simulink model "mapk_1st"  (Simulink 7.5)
settings: Solver=ode45  StartTime=0.0  StopTime=1000  FixedStep=0.001  RelTol=1e-3
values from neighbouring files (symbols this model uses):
  k = load('parameter.txt', '-ascii')    [mapk_steering.m]
  x = xis+deltax    [mapk_steering.m]

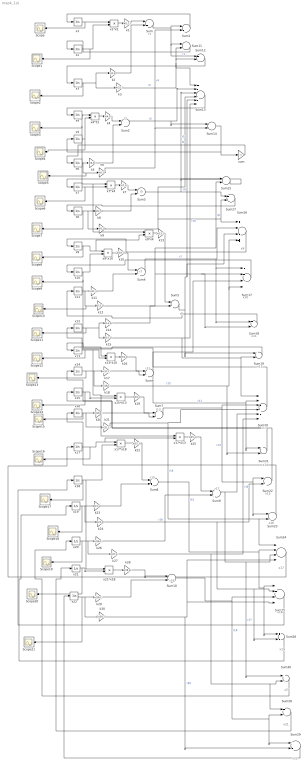
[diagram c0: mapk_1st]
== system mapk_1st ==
  note: r3
  note: r5
  note: r7
  note: r9
  note: r11
  note: r13
  note: r15
  note: r17
  note: r19
  note: x9
  note: x10
  note: x11
  note: x12
  note: x13
  note: x14
  note: x15
  note: x16
  note: x17
  note: x18
  note: x19
  note: x20
  note: x21
  note: x22
  note: r1
  Scope{,1..21} (22 alike) : Scope
  Sum{,2..10} (10 alike) : Sum  Inputs=|+-  OutDataType=fixdt(1, 16)  OutScaling=2^0
  Sum{1,11,14..15} (4 alike) : Sum  Inputs=|-+  OutDataType=fixdt(1, 16)  OutScaling=2^0
  Sum{12,18..19,21,23,26..30} (10 alike) : Sum  Inputs=+-  OutDataType=fixdt(1, 16)  OutScaling=2^0
  Sum13 : Sum  Inputs=+--+-+  OutDataType=fixdt(1, 16)  OutScaling=2^0
  Sum16 : Sum  Inputs=+--+  OutDataType=fixdt(1, 16)  OutScaling=2^0
  Sum17 : Sum  Inputs=-+-+  OutDataType=fixdt(1, 16)  OutScaling=2^0
  Sum20 : Sum  Inputs=+--+-+  OutDataType=fixdt(1, 16)  OutScaling=2^0
  Sum22 : Sum  Inputs=-+  OutDataType=fixdt(1, 16)  OutScaling=2^0
  Sum24 : Sum  Inputs=+--+  OutDataType=fixdt(1, 16)  OutScaling=2^0
  Sum25 : Sum  Inputs=-+-+  OutDataType=fixdt(1, 16)  OutScaling=2^0
  k1 : Gain  Gain=k(1,1)  ParameterDataType=fixdt(1, 16)  ParameterScaling=2^0  OutDataType=fixdt(1, 16)  OutScaling=2^0
  k10 : Gain  Gain=k(10,1)  ParameterDataType=fixdt(1, 16)  ParameterScaling=2^0  OutDataType=fixdt(1, 16)  OutScaling=2^0
  k11 : Gain  Gain=k(11,1)  ParameterDataType=fixdt(1, 16)  ParameterScaling=2^0  OutDataType=fixdt(1, 16)  OutScaling=2^0
  k12 : Gain  Gain=k(12,1)  ParameterDataType=fixdt(1, 16)  ParameterScaling=2^0  OutDataType=fixdt(1, 16)  OutScaling=2^0
  k13 : Gain  Gain=k(13,1)  ParameterDataType=fixdt(1, 16)  ParameterScaling=2^0  OutDataType=fixdt(1, 16)  OutScaling=2^0
  k14 : Gain  Gain=k(14,1)  ParameterDataType=fixdt(1, 16)  ParameterScaling=2^0  OutDataType=fixdt(1, 16)  OutScaling=2^0
  k15 : Gain  Gain=k(15,1)  ParameterDataType=fixdt(1, 16)  ParameterScaling=2^0  OutDataType=fixdt(1, 16)  OutScaling=2^0
  k16 : Gain  Gain=k(16,1)  ParameterDataType=fixdt(1, 16)  ParameterScaling=2^0  OutDataType=fixdt(1, 16)  OutScaling=2^0
  k17 : Gain  Gain=k(17,1)  ParameterDataType=fixdt(1, 16)  ParameterScaling=2^0  OutDataType=fixdt(1, 16)  OutScaling=2^0
  k18 : Gain  Gain=k(18,1)  ParameterDataType=fixdt(1, 16)  ParameterScaling=2^0  OutDataType=fixdt(1, 16)  OutScaling=2^0
  k19 : Gain  Gain=k(19,1)  ParameterDataType=fixdt(1, 16)  ParameterScaling=2^0  OutDataType=fixdt(1, 16)  OutScaling=2^0
  k2 : Gain  Gain=k(2,1)  ParameterDataType=fixdt(1, 16)  ParameterScaling=2^0  OutDataType=fixdt(1, 16)  OutScaling=2^0
  k20 : Gain  Gain=k(20,1)  ParameterDataType=fixdt(1, 16)  ParameterScaling=2^0  OutDataType=fixdt(1, 16)  OutScaling=2^0
  k21 : Gain  Gain=k(21,1)  ParameterDataType=fixdt(1, 16)  ParameterScaling=2^0  OutDataType=fixdt(1, 16)  OutScaling=2^0
  k22 : Gain  Gain=k(22,1)  ParameterDataType=fixdt(1, 16)  ParameterScaling=2^0  OutDataType=fixdt(1, 16)  OutScaling=2^0
  k23 : Gain  Gain=k(23,1)  ParameterDataType=fixdt(1, 16)  ParameterScaling=2^0  OutDataType=fixdt(1, 16)  OutScaling=2^0
  k24 : Gain  Gain=k(24,1)  ParameterDataType=fixdt(1, 16)  ParameterScaling=2^0  OutDataType=fixdt(1, 16)  OutScaling=2^0
  k25 : Gain  Gain=k(25,1)  ParameterDataType=fixdt(1, 16)  ParameterScaling=2^0  OutDataType=fixdt(1, 16)  OutScaling=2^0
  k26 : Gain  Gain=k(26,1)  ParameterDataType=fixdt(1, 16)  ParameterScaling=2^0  OutDataType=fixdt(1, 16)  OutScaling=2^0
  k27 : Gain  Gain=k(27,1)  ParameterDataType=fixdt(1, 16)  ParameterScaling=2^0  OutDataType=fixdt(1, 16)  OutScaling=2^0
  k28 : Gain  Gain=k(28,1)  ParameterDataType=fixdt(1, 16)  ParameterScaling=2^0  OutDataType=fixdt(1, 16)  OutScaling=2^0
  k29 : Gain  Gain=k(29,1)  ParameterDataType=fixdt(1, 16)  ParameterScaling=2^0  OutDataType=fixdt(1, 16)  OutScaling=2^0
  k3 : Gain  Gain=k(3,1)  ParameterDataType=fixdt(1, 16)  ParameterScaling=2^0  OutDataType=fixdt(1, 16)  OutScaling=2^0
  k30 : Gain  Gain=k(30,1)  ParameterDataType=fixdt(1, 16)  ParameterScaling=2^0  OutDataType=fixdt(1, 16)  OutScaling=2^0
  k4 : Gain  Gain=k(4,1)  ParameterDataType=fixdt(1, 16)  ParameterScaling=2^0  OutDataType=fixdt(1, 16)  OutScaling=2^0
  k5 : Gain  Gain=k(5,1)  ParameterDataType=fixdt(1, 16)  ParameterScaling=2^0  OutDataType=fixdt(1, 16)  OutScaling=2^0
  k6 : Gain  Gain=k(6,1)  ParameterDataType=fixdt(1, 16)  ParameterScaling=2^0  OutDataType=fixdt(1, 16)  OutScaling=2^0
  k7 : Gain  Gain=k(7,1)  ParameterDataType=fixdt(1, 16)  ParameterScaling=2^0  OutDataType=fixdt(1, 16)  OutScaling=2^0
  k8 : Gain  Gain=k(8,1)  ParameterDataType=fixdt(1, 16)  ParameterScaling=2^0  OutDataType=fixdt(1, 16)  OutScaling=2^0
  k9 : Gain  Gain=k(9,1)  ParameterDataType=fixdt(1, 16)  ParameterScaling=2^0  OutDataType=fixdt(1, 16)  OutScaling=2^0
  sum : Gain  Gain=-1  ParameterDataType=fixdt(1, 16)  ParameterScaling=2^0  OutDataType=fixdt(1, 16)  OutScaling=2^0
  x1 : Integrator  InitialCondition=x(1,1)  LimitOutput=on  LowerSaturationLimit=0
  x1*x2 : Product  OutDataType=fixdt(1, 16)  OutScaling=2^0
  x10 : Integrator  InitialCondition=x(10,1)  LimitOutput=on  LowerSaturationLimit=0
  x11 : Integrator  InitialCondition=x(11,1)  LimitOutput=on  LowerSaturationLimit=0
  x12 : Integrator  InitialCondition=x(12,1)  LimitOutput=on  LowerSaturationLimit=0
  x13 : Integrator  InitialCondition=x(13,1)  LimitOutput=on  LowerSaturationLimit=0
  x13*x10 : Product  OutDataType=fixdt(1, 16)  OutScaling=2^0
  x14 : Integrator  InitialCondition=x(14,1)  LimitOutput=on  LowerSaturationLimit=0
  x15 : Integrator  InitialCondition=x(15,1)  LimitOutput=on  LowerSaturationLimit=0
  x15*x13 : Product  OutDataType=fixdt(1, 16)  OutScaling=2^0
  x16 : Integrator  InitialCondition=x(16,1)  LimitOutput=on  LowerSaturationLimit=0
  x17 : Integrator  InitialCondition=x(17,1)  LimitOutput=on  LowerSaturationLimit=0
  x17*x13 : Product  OutDataType=fixdt(1, 16)  OutScaling=2^0
  x17*x18 : Product  OutDataType=fixdt(1, 16)  OutScaling=2^0
  x18 : Integrator  InitialCondition=x(18,1)  LimitOutput=on  LowerSaturationLimit=0
  x19 : Integrator  InitialCondition=x(19,1)  LimitOutput=on  LowerSaturationLimit=0
  x2 : Integrator  InitialCondition=x(2,1)  LimitOutput=on  LowerSaturationLimit=0
  x20 : Integrator  InitialCondition=x(20,1)  LimitOutput=on  LowerSaturationLimit=0
  x21 : Integrator  InitialCondition=x(21,1)  LimitOutput=on  LowerSaturationLimit=0
  x21*x18 : Product  OutDataType=fixdt(1, 16)  OutScaling=2^0
  x22 : Integrator  InitialCondition=x(22,1)  LimitOutput=on  LowerSaturationLimit=0  ZeroCross=off
  x3 : Integrator  InitialCondition=x(3,1)  LimitOutput=on  LowerSaturationLimit=0
  x4 : Integrator  InitialCondition=x(4,1)  LimitOutput=on  LowerSaturationLimit=0
  x4*51 : Product  OutDataType=fixdt(1, 16)  OutScaling=2^0
  x5 : Integrator  InitialCondition=x(5,1)  LimitOutput=on  LowerSaturationLimit=0
  x6 : Integrator  InitialCondition=x(6,1)  LimitOutput=on  LowerSaturationLimit=0
  x7 : Integrator  InitialCondition=x(7,1)  LimitOutput=on  LowerSaturationLimit=0
  x7*x4 : Product  OutDataType=fixdt(1, 16)  OutScaling=2^0
  x8 : Integrator  InitialCondition=x(8,1)  LimitOutput=on  LowerSaturationLimit=0
  x9 : Integrator  InitialCondition=x(9,1)  LimitOutput=on  LowerSaturationLimit=0
  x9*x10 : Product  OutDataType=fixdt(1, 16)  OutScaling=2^0
  x9*x4 : Product  OutDataType=fixdt(1, 16)  OutScaling=2^0
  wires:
  x2/1 -> Scope1/1, x1*x2/2
  x3/1 -> k2/1, k3/1, Scope2/1
  k2/1 -> Sum/2
  x4/1 -> x4*51/1, x7*x4/1, x9*x4/1, Scope3/1
  x5/1 -> x4*51/2, Scope4/1
  x4*51/1 -> k4/1
  x6/1 -> k6/1, Scope5/1, k5/1
  k4/1 -> Sum2/1
  k5/1 -> Sum2/2
  x7/1 -> x7*x4/2, Scope6/1
  x7*x4/1 -> k7/1
  x8/1 -> k8/1, k9/1, Scope7/1
  k7/1 -> Sum3/1
  k8/1 -> Sum3/2
  x9/1 -> x9*x10/1, x9*x4/2, Scope8/1
  x10/1 -> x9*x10/2, x13*x10/1, Scope9/1
  x9*x10/1 -> k10/1
  x11/1 -> k11/1, k12/1, Scope10/1
  k10/1 -> Sum4/1
  k11/1 -> Sum4/2
  x9*x4/1 -> k13/1
  k13/1 -> Sum5/1
  x12/1 -> k14/1, k15/1, Scope11/1
  k14/1 -> Sum5/2
  x13*x10/1 -> k16/1
  x13/1 -> x13*x10/2, x15*x13/1, x17*x13/1, Scope12/1
  x14/1 -> k17/1, k18/1, Scope13/1
  k16/1 -> Sum6/1
  k17/1 -> Sum6/2
  x15/1 -> x15*x13/2, Scope14/1
  x15*x13/1 -> k19/1
  x16/1 -> k20/1, k21/1, Scope15/1
  k19/1 -> Sum7/1
  k20/1 -> Sum7/2
  x17/1 -> x17*x18/1, x17*x13/2, Scope16/1
  x18/1 -> x17*x18/2, x21*x18/1, Scope17/1
  x17*x18/1 -> k22/1
  x19/1 -> k23/1, k24/1, Scope18/1
  k22/1 -> Sum8/1
  k23/1 -> Sum8/2
  x17*x13/1 -> k25/1
  k25/1 -> Sum9/1
  x20/1 -> k26/1, k27/1, Scope19/1
  k26/1 -> Sum9/2
  x22/1 -> k29/1, k30/1, Scope21/1
  x21/1 -> x21*x18/2, Scope20/1
  x21*x18/1 -> k28/1
  k28/1 -> Sum10/1
  k29/1 -> Sum10/2
  k6/1 -> Sum14/2, Sum1/2  "r4"
  k3/1 -> Sum11/2, Sum12/2, Sum13/1  "r2"
  Sum2/1 -> Sum13/2, Sum14/1  "r3"
  Sum3/1 -> Sum13/3, Sum15/1, Sum27/1  "r5"
  k9/1 -> Sum13/4, Sum16/1, Sum27/2  "r6"
  k15/1 -> Sum13/6, Sum19/2, Sum20/1  "r10"
  Sum5/1 -> Sum13/5, Sum16/3, Sum19/1  "r9"
  Sum14/1 -> sum/1, x5/1
  k12/1 -> Sum15/2, Sum17/2, Sum18/2  "r8"
  Sum15/1 -> x7/1
  Sum4/1 -> Sum16/2, Sum17/1, Sum18/1  "r7"
  k18/1 -> Sum16/4, Sum17/4, Sum21/2  "r12"
  Sum6/1 -> Sum17/3, Sum20/2, Sum21/1  "r11"
  Sum7/1 -> Sum20/3, Sum22/1, Sum23/1  "r13"
  k21/1 -> Sum20/4, Sum23/2, Sum24/1  "r14"
  Sum9/1 -> Sum20/5, Sum24/3, Sum30/1  "r17"
  k27/1 -> Sum20/6, Sum30/2, Sum28/1  "r18"
  k24/1 -> Sum22/2, Sum25/2, Sum26/2  "r16"
  Sum8/1 -> Sum24/2, Sum25/1, Sum26/1  "r15"
  k30/1 -> Sum24/4, Sum25/4, Sum29/2  "r20"
  Sum10/1 -> Sum25/3, Sum28/2, Sum29/1  "r19"
  Sum12/1 -> x3/1
  Sum13/1 -> x4/1
  sum/1 -> x6/1
  Sum29/1 -> x22/1
  Sum28/1 -> x21/1
  Sum30/1 -> x20/1
  Sum26/1 -> x19/1
  Sum25/1 -> x18/1
  Sum24/1 -> x17/1
  Sum23/1 -> x16/1
  Sum22/1 -> x15/1
  Sum21/1 -> x14/1
  Sum20/1 -> x13/1
  Sum19/1 -> x12/1
  Sum18/1 -> x11/1
  Sum17/1 -> x10/1
  Sum16/1 -> x9/1
  Sum27/1 -> x8/1
  Sum11/1 -> x2/1
  x1/1 -> x1*x2/1, Scope/1
  x1*x2/1 -> k1/1
  k1/1 -> Sum/1
  Sum1/1 -> x1/1
  Sum/1 -> Sum1/1, Sum11/1, Sum12/1  "r1"
